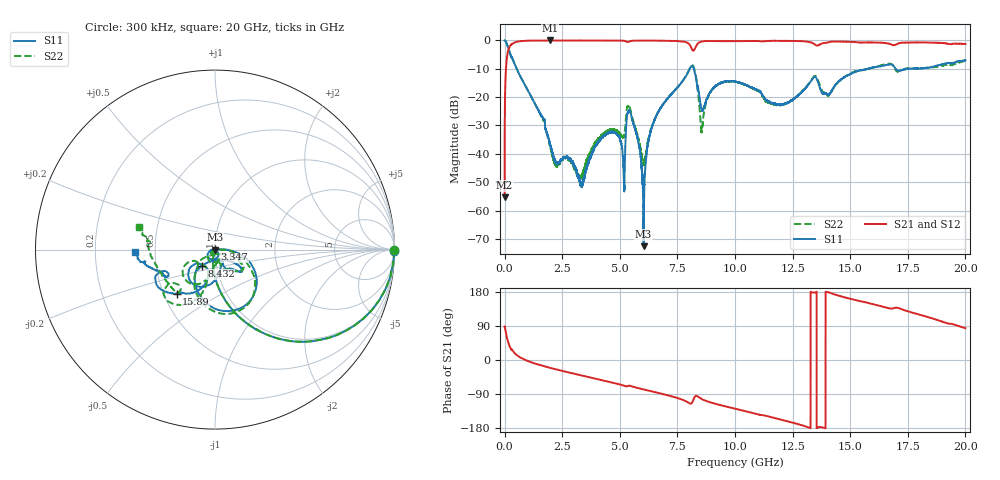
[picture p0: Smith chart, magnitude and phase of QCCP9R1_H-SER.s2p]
!{QCCP9R1}
!Johanson Technology Inc.
!www.johansontechnology.com
!Test Board Conditions:
!Substrate Type  RO4350B
!Substrate Thickness  20 mil
!Substrate Dk  3.66
!TL Type: GCPW
!TL Trace Width  36 mil
!TL Gap  12 mil
!Electrode orientation  Horizontal
!DUT TOPOLOGY	SERIES
!Mounting Pad LxW  26x36 mil
! Created Sat Jan  9 18:31:27 2021
# hz S ma R 50
! 2 Port Network Data from SP1.SP block
! freq  magS11  angS11  magS21  angS21  magS12  angS12  magS22  angS22
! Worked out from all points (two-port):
!   20001 points, 300 kHz to 20 GHz, reference 50 ohm
!   highest |S21| = -0.01 dB at 1.971 GHz (marker M1); lowest = -55.3 dB at 300 kHz (marker M2)
!   |S21| within 3 dB of the highest: 176.5 MHz to 8.128 GHz (7.952 GHz wide, 191 % of centre); 8.251 GHz to end of sweep
!   lowest |S11| = -72.6 dB at 6.033 GHz (marker M3), VSWR 1.00, Z = 50 + j0.0222 ohm
!   |S11| at or under -10 dB: 524.6 MHz to 8.038 GHz (7.514 GHz wide, 175 % of centre); 8.216 GHz to 15.76 GHz (7.548 GHz wide, 63 % of centre); 16.98 GHz to 17.5 GHz (528.4 MHz wide, 3.06 % of centre)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
!   |S22| runs from -48.8 to 0.0 dB; largest |S21 - S12| = 0.018
!   S11 on the Smith chart (normalised r, x): 300 kHz: open; 3.347 GHz: 1.00, +0.01; 8.432 GHz: 0.85, -0.16; 15.89 GHz: 0.58, -0.32; 20 GHz: 0.38, -0.01
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300000  1 -0.3  0.001718 87.9  0.001706 89.5  0.9996 -0.2
1.053e8  0.8561 -32.1  0.512 57.8  0.5131 57.7  0.8567 -32.0
2.253e8  0.6089 -54.5  0.7882 35.2  0.788 35.1  0.6099 -54.4
1.9713e9  0.01512 -83.4  0.9985 -20.6  0.998 -20.6  0.0137 -137.1
3.3343e9  0.002874 101.1  0.9969 -40.7  0.9959 -40.7  0.003893 -15.4
3.3473e9  0.002686 102.8  0.9967 -40.9  0.9962 -40.9  0.003884 -20.4
4.4983e9  0.02335 -171.5  0.9955 -57.2  0.9957 -57.1  0.02587 -117.1
5.1563e9  0.006309 -172.0  0.9894 -67.2  0.989 -67.2  0.01997 -87.3
5.4063e9  0.059 -117.8  0.9515 -67.9  0.9504 -67.9  0.07179 -112.2
6.0333e9  0.0002349 109.3  0.9929 -77.7  0.9943 -77.6  0.006533 -79.0
6.6673e9  0.05459 0.0  0.992 -86.9  0.9914 -86.9  0.05449 -0.7
8.1213e9  0.3559 -64.1  0.7175 -114.0  0.7162 -113.7  0.3654 -66.3
8.4323e9  0.1184 -129.2  0.9166 -98.4  0.9172 -98.3  0.08635 -144.1
8.5763e9  0.05748 -86.9  0.9613 -103.6  0.9627 -103.6  0.02753 -60.9
8.9883e9  0.1327 -34.5  0.9755 -112.8  0.9767 -112.8  0.1336 -24.2
1.00003e10  0.1884 -40.6  0.9733 -128.5  0.9719 -128.5  0.1851 -39.2
1.19003e10  0.07422 -57.2  0.9845 -155.9  0.9868 -155.9  0.07373 -76.5
1.33343e10  0.2022 -100.9  0.9117 178.8  0.916 178.7  0.2058 -113.5
1.40673e10  0.1104 -117.1  0.9323 178.5  0.9334 178.4  0.1072 -123.8
1.58913e10  0.3253 -131.1  0.9219 148.7  0.9266 148.7  0.3257 -114.2
1.66673e10  0.374 -144.7  0.8791 136.7  0.8706 136.5  0.388 -131.2
2e10  0.4469 -178.2  0.8673 84.1  0.8563 83.9  0.445 162.9
